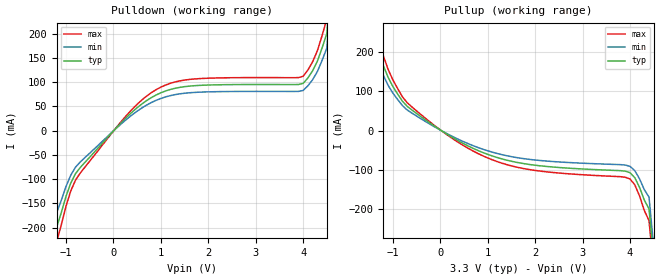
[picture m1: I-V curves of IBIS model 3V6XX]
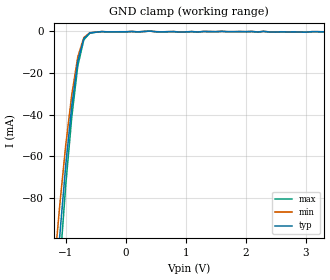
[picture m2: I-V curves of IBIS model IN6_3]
[IBIS Ver]   2.1
[File name]   524_3.ibs
[File Rev]   2.1
[Date]   8/30/06
[Source]   ICS MicroClock Applications Engineering
[Disclaimer] This information is for modeling purposes only, and is
   not guaranteed.
(C) Copyright Integrated Circuit Systems, Inc. 1997-2001
   All rights reserved
ICS hereby grants the user of this IBIS model a non-exclusive,
nontransferable license to use this IBIS model under the following terms.
Before using this IBIS model, the user should read this license.
If the user does not accept these terms,  the IBIS model should be
returned to ICS within 30 days.
   The user is granted this license only to use the IBIS model and
is not granted rights to sell, load, rent, lease or license the IBIS
model in whole or in part, or in modified form to anyone other than
user. User may modify the IBIS model to suit its specific
applications but rights to derivative works and such modifications
shall belong to ICS.
   This IBIS model is provided on an "AS IS" basis and ICS makes
absolutely no warranty with respect to the information contained
herein. ICS DISCLAIMS AND CUSTOMER WAIVES ALL WARRANTIES, EXPRESS
OR IMPLIED, INCLUDING WARRANTIES OF MERCHANTABILITY OR FITNESS FOR
A PARTICULAR PURPOSE. The entire risk as to quality and performance
is with the Customer. ACCORDINGLY, IN NO EVENT SHALL THE COMPANY BE
LIABLE FOR ANY DAMAGES, WHETHER IN CONTRACT OR TORT,INCLUDING ANY
LOST PROFITS OR OTHER INCIDENTAL, CONSEQUENTIAL, EXEMPLARY, OR
PUNITIVE DAMAGES ARISING OUT OF THE USE OR APPLICATION OF THE IBIS
model provided in this package. Further, ICS reserves the right to
make changes without notice to any product herein to improve
reliability, function, or design. ICS does not convey any license
under patent rights or any other intellectual property rights,
including those of third parties.
   ICS is not obligated to provide maintenance or support
for the licensed IBIS model.
[Component]   ICS524
[Manufacturer] Integrated Circuit Systems Inc.
[Package]
|   typ   min   max
R_pkg   40m   35m   45m
L_pkg   1.65nH   1.35nH   1.95nH
C_pkg   0.24pF   0.14pF   0.34pF
[pin]   signal_name   model_name   R_pin   L_pin   C_pin
   1   ICLK   IN6_3   58.6m   1.968nH   0.286pF
   2   Q0   3V6XX   55.5m   1.570nH   0.252pF
   3   Q1   3V6XX   55.5m   1.570nH   0.252pF
   4   NC   NC
   5   VDD   POWER
   6   Q2   3V6XX   55.5m   1.570nH   0.252pF
   7   Q3   3V6XX   55.5m   1.570nH   0.252pF
   8   GND   GND
| Models and submodels in the file (2): 3V6XX (Output), IN6_3 (Input)
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|   ICS524 3.3V Clock Drive Model
| This model is suitable for all output pins on the
|  ICS524
[Model]   3V6XX
Model_type   Output
Polarity   Non-Inverting
Vmeas=1.65V
|   typ   min   max
C_comp   5pF   4pF   6pF
|   typ   min   max
[Voltage range]  3.3V   3.15V   3.45V
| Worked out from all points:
|   slope of the pulldown table from 0 to 0.495 V, typ, clamps not added: 10.4 ohm
|   slope of the pullup table from 0 to 0.495 V, typ, clamps not added: 14 ohm
[pulldown]
|Voltage I (typ)   I (min)   I (max)
-3.3V     -3A        -3A        -3A
-1.2V     -200.1mA   -170mA     -230.1mA
-1.1V     -169.4mA   -144mA     -194.8mA
-900mV    -108.4mA   -92.1mA    -124.6mA
-700mV    -76.24mA   -64.8mA    -87.68mA
400mV     38.57mA    32.79mA    44.36mA
1.1V      81.57mA    69.34mA    93.81mA
1.8V      92.97mA    79.03mA    106.9mA
4V        97.22mA    82.64mA    111.8mA
4.3V      143.1mA    121.7mA    164.6mA
4.5V      200.3mA    170.3mA    230.3mA
6.6V      3A         3A         3A
[pullup]
|Voltage I (typ)   I (min)   I (max)
-3.3V     3A         3A         3A
-1.3V     200.3mA    170.2mA    230.3mA
-1.1V     135.6mA    115.3mA    156mA
-1V       112.4mA    95.55mA    129.3mA
-700mV    61.99mA    52.69mA    71.29mA
200mV     -13.76mA   -11.69mA   -15.82mA
900mV     -56.35mA   -47.89mA   -64.8mA
1.9V      -87.07mA   -74.01mA   -100.1mA
4V        -107.7mA   -91.55mA   -123.9mA
4.1V      -120.5mA   -102.4mA   -138.6mA
4.4V      -200.1mA   -170.1mA   -230.1mA
6.6V      -3A        -3A        -3A
[Ramp]
|   typ   min   max
dV/dt_r   1.56/0.36n   1.48/0.40n   1.64/0.32n
dV/dt_f   1.65/0.32n   1.57/0.35n   1.73/0.29n
|   3.3V  INPUT  Model
| This model is suitable for ALL INPUT Pin
[Model]   IN6_3
Model_type   Input
Polarity   Non-Inverting
Vinl = 1.15V   | input logic "low" DC voltage
Vinh = 2.15V   | input logic "high" DC voltage
|   typ   min   max
C_comp   5pF   4pF   6pF
|   typ   min   max
[Voltage range]  3.3V   2.97V   3.63V
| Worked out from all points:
|   GND clamp passes 1 mA (typ) near -0.61 V on its own axis
[GND_clamp]
|Voltage I (typ)   I (min)   I (max)
-3.3V     -3A        -3A        -3A
-1.2V     -135.8mA   -115.4mA   -156.1mA
-1.1V     -97.7mA    -83.05mA   -112.4mA
-1V       -63.72mA   -54.16mA   -73.28mA
-900mV    -35.55mA   -30.22mA   -40.89mA
-800mV    -14.29mA   -12.15mA   -16.44mA
-700mV    -3.48mA    -2.958mA   -4.002mA
-600mV    -708uA     -601.8uA   -814.2uA
-400mV    -72.3uA    -61.47uA   -83.16uA
400mV     155uA      131.8uA    178.2uA
900mV     -299uA     -254.2uA   -343.8uA
3.3V      -163uA     -138.6uA   -187.5uA
